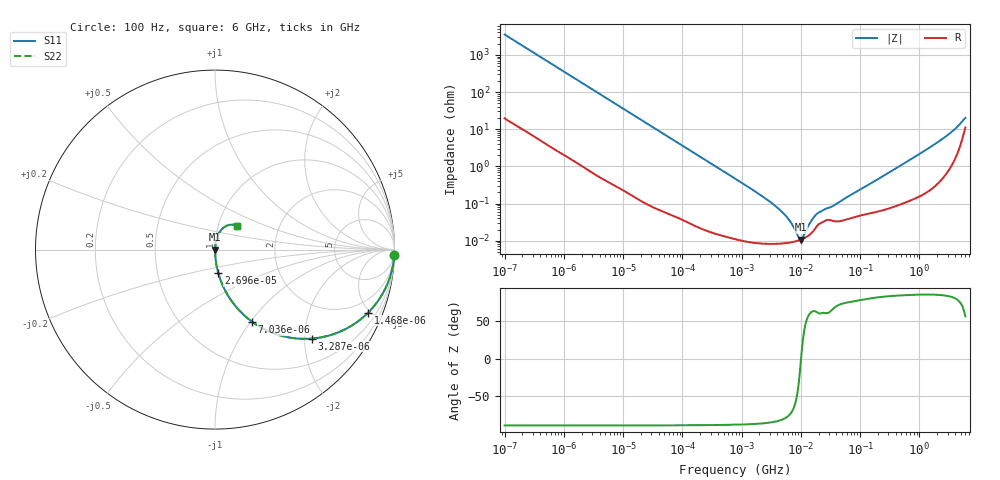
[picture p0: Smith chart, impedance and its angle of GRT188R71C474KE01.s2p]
!Murata Part Number: GRT188R71C474KE01
!These Parameters are Measured in Series Mode Connection
!Data Generated on Jun 19, 2026
!  o--ll--o
!Port1  Port2
!  o------o
!Operation Temp=25[degC], DC Bias Voltage=0[V]
!Freq. Start=100[Hz] Stop=6[GHz] 401[Steps]
# Hz S RI R 50
!Freq.(Hz) S11(Real) S11(Imag) S21(Real) S21(Imag) S12(Real) S12(Imag) S22(Real) S22(Imag)
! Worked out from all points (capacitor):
!   401 points, 100 Hz to 6 GHz, reference 50 ohm
!   read as one part in series: C = 451 nF near 109 Hz
!   lowest |Z| = 10.7 mohm at 9.942 MHz (marker M1)
!   series resonance near 10.09 MHz, so ESL is about 550 pH
!   S11 on the Smith chart (normalised r, x): 100 Hz: 1, -71; 1.468 kHz: 1.03, -4.85; 3.287 kHz: 1.01, -2.17; 7.036 kHz: 1.01, -1.02; 26.96 kHz: 1.00, -0.27; 6 GHz: 1.22, +0.34
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100  0.999 -0.0283  0.00096 0.0283  0.00096 0.0283  0.999 -0.0283
438  0.9843 -0.1216  0.0157 0.1216  0.0157 0.1216  0.9843 -0.1216
1468  0.8533 -0.351  0.1467 0.351  0.1467 0.351  0.8533 -0.351
2008  0.7578 -0.4256  0.2422 0.4256  0.2422 0.4256  0.7578 -0.4256
3287  0.5411 -0.4955  0.4589 0.4955  0.4589 0.4955  0.5411 -0.4955
7036  0.2071 -0.4022  0.7929 0.4022  0.7929 0.4022  0.2071 -0.4022
12592  0.0765 -0.2627  0.9235 0.2627  0.9235 0.2627  0.0765 -0.2627
26957  0.0184 -0.1309  0.9816 0.1309  0.9816 0.1309  0.0184 -0.1309
40335  0.00857 -0.0885  0.9914 0.0885  0.9914 0.0885  0.00857 -0.0885
774597  0.000132 -0.0047  0.9999 0.0047  0.9999 0.0047  0.000132 -0.0047
4440638  8.37e-05 -0.000669  0.9999 0.000669  0.9999 0.000669  8.37e-05 -0.000669
6353432  8.86e-05 -0.000351  0.9999 0.000351  0.9999 0.000351  8.86e-05 -0.000351
9090158  0.000101 -7.69e-05  0.9999 7.69e-05  0.9999 7.69e-05  0.000101 -7.69e-05
9941735  0.000106 -1.11e-05  0.9999 1.11e-05  0.9999 1.11e-05  0.000106 -1.11e-05
1.087309e7  0.000113 5.49e-05  0.9999 -5.49e-05  0.9999 -5.49e-05  0.000113 5.49e-05
1.555665e7  0.000168 0.000332  0.9998 -0.000332  0.9998 -0.000332  0.000168 0.000332
2.035112e7  0.000283 0.000504  0.9997 -0.000504  0.9997 -0.000504  0.000283 0.000504
3.64232e7  0.000335 0.000827  0.9997 -0.000827  0.9997 -0.000827  0.000335 0.000827
3.124326e8  0.00079 0.00687  0.9992 -0.00687  0.9992 -0.00687  0.00079 0.00687
2.240541e9  0.00633 0.0488  0.9937 -0.0488  0.9937 -0.0488  0.00633 0.0488
4.193612e9  0.0288 0.1016  0.9712 -0.1016  0.9712 -0.1016  0.0288 0.1016
6e9  0.1202 0.1334  0.8798 -0.1334  0.8798 -0.1334  0.1202 0.1334
